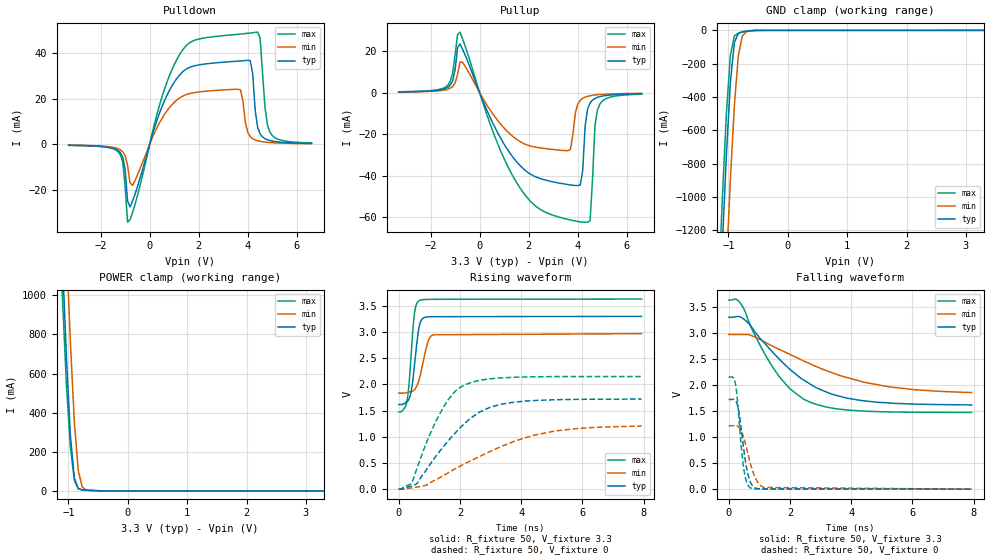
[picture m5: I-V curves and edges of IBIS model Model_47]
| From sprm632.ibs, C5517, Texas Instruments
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| Model based on original model for BC3350CTHYPU
|   Sub model PU_ON_COM_3P3
[model]   Model_47
|[Description]  [3.3V-I/O-PU-X, COM]
|   PU,COM,
|[Input Load]   PU
|[Output Drive]
|Voltage   3.3V
|Mode   I/O
Model_type   I/O
Polarity   Non-Inverting
Enable   Active-Low
Vinl =  0.8
Vinh =  2
Cref =  15.0000pF
Rref =  100.0000M
Vref =  0V
Vmeas =  1.65
C_comp   0.87673039p  0.86952386p   1.2993811p
[Model Spec]
Vinl   0.8   0.8   0.8
Vinh   2   2   2
[Temperature Range]   25   105   -10
[Voltage Range]   3.3   2.97   3.63
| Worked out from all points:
|   slope of the pulldown table from 0 to 0.495 V, typ, clamps not added: 30.2 ohm
|   slope of the pullup table from 0 to 0.495 V, typ, clamps not added: 36.2 ohm
|   GND clamp passes 1 mA (typ) near -0.58 V on its own axis
|   POWER clamp passes 1 mA (typ) near -0.52 V on its own axis
|   rising waveform, R_fixture 50, V_fixture 3.3: 20-80 % time 198ps typ, 268ps min, 165ps max; typ from 1.62 V to 3.3 V
|   rising waveform, R_fixture 50, V_fixture 0: 20-80 % time 1.53ns typ, 2.64ns min, 1.02ns max; typ from 0.002 V to 1.72 V
|   falling waveform, R_fixture 50, V_fixture 3.3: 20-80 % time 1.91ns typ, 2.84ns min, 1.38ns max; typ from 3.3 V to 1.62 V
|   falling waveform, R_fixture 50, V_fixture 0: 20-80 % time 244ps typ, 350ps min, 199ps max; typ from 1.72 V to 0.002 V
[POWER_clamp]
-3.3V     22.37A     22.96A     22.14A
-1.167V   1.737A     2.381A     1.512A
-1.1V     1.183A     1.806A     986.6mA
-1.033V   682.1mA    1.26A      542.1mA
-966.7mV  284.5mA    761.6mA    224.8mA
-900mV    65.81mA    352.3mA    53.51mA
-833.3mV  11.58mA    102.8mA    10.59mA
-766.7mV  4.716mA    20.06mA    5.567mA
-700mV    3.207mA    4.896mA    4.024mA
-633.3mV  2.25mA     2.24mA     2.841mA
3.3V      -103.5uA   -77.89uA   -144.3uA
[Pulldown]
-3.3V     -379.4uA   -332.5uA   -410.9uA
-1.2V     -3.537mA   -2.351mA   -4.45mA
-1V       -10.99mA   -4.979mA   -18.19mA
-900mV    -24.8mA    -9.223mA   -34.14mA
-700mV    -24.92mA   -18.03mA   -29.99mA
500mV     16.51mA    11.37mA    20.75mA
1.5V      33.12mA    21.9mA     43.48mA
3.7V      36.65mA    23.93mA    48.44mA
4.1V      36.79mA    3.426mA    48.89mA
4.4V      7.557mA    1.597mA    49.31mA
4.9V      1.707mA    822.5uA    5.402mA
6.6V      436uA      304.4uA    625.7uA
[Pullup]
-3.3V     352.6uA    285.2uA    404.5uA
-1.3V     2.559mA    1.632mA    3.524mA
-800mV    23.47mA    14.67mA    29.18mA
800mV     -20.79mA   -14.38mA   -26.49mA
2V        -38.75mA   -25.51mA   -51.47mA
3.7V      -44.51mA   -27.32mA   -61.38mA
4.2V      -37.5mA    -2.71mA    -62.46mA
4.3V      -15.99mA   -2.138mA   -62.46mA
4.5V      -4.997mA   -1.493mA   -61.74mA
4.7V      -2.803mA   -1.142mA   -15.75mA
4.9V      -1.928mA   -922.7uA   -5.515mA
6.6V      -515.4uA   -347uA     -755.5uA
[GND_clamp]
-3.3V     -22.52A    -23.16A    -22.27A
-1.167V   -1.839A    -2.548A    -1.554A
-1.1V     -1.269A    -1.966A    -993.7mA
-1.033V   -744.2mA   -1.409A    -496.6mA
-966.7mV  -312.7mA   -893.3mA   -149.2mA
-900mV    -73.61mA   -452.5mA   -34.27mA
-833.3mV  -18.5mA    -154mA     -16.8mA
-766.7mV  -8.937mA   -34.95mA   -10.26mA
-700mV    -4.785mA   -8.919mA   -5.557mA
-633.3mV  -2.174mA   -3.321mA   -2.412mA
3.3V      469pA      103.6uA    -29.49uA
[Ramp]
dV/dt_f  1.0208248/1.9222786n 0.68955168/2.9572302n  1.3051325/1.3845332n
dV/dt_r  1.0324428/1.5316798n 0.73040027/2.6850092n  1.2903206/1.0171168n
R_load = 50
[Rising Waveform]
R_fixture = 50
V_fixture = 3.3
V_fixture_min = 2.97
V_fixture_max = 3.63
0s        1.617V     1.835V     1.475V
258.2ps   1.665V     1.845V     1.646V
316.8ps   1.7V       1.852V     1.878V
381.2ps   1.797V     1.861V     2.348V
469.6ps   2.119V     1.879V     3.082V
523.7ps   2.41V      1.906V     3.389V
692.9ps   3.16V      2.15V      3.606V
955.9ps   3.29V      2.814V     3.624V
1.128ns   3.294V     2.948V     3.625V
7.933ns   3.3V       2.97V      3.63V
[Rising Waveform]
R_fixture = 50
V_fixture = 0
V_fixture_min = 0
V_fixture_max = 0
0s        2.331mV    2.258mV    2.773mV
416.9ps   60.92mV    27.58mV    119mV
604.9ps   116.9mV    43.18mV    412.1mV
1.347ns   731.5mV    223.8mV    1.445V
1.792ns   1.04V      373.7mV    1.838V
2.183ns   1.272V     493.9mV    1.998V
3.005ns   1.57V      726.5mV    2.109V
3.777ns   1.662V     915.7mV    2.138V
5.109ns   1.709V     1.112V     2.15V
7.933ns   1.721V     1.206V     2.152V
[Falling Waveform]
R_fixture = 50
V_fixture = 3.3
V_fixture_min = 2.97
V_fixture_max = 3.63
0s        3.3V       2.97V      3.63V
376.7ps   3.309V     2.97V      3.576V
903.3ps   2.983V     2.907V     2.9V
1.423ns   2.639V     2.747V     2.356V
1.986ns   2.306V     2.592V     1.934V
2.534ns   2.065V     2.439V     1.703V
3.338ns   1.83V      2.244V     1.561V
4.328ns   1.702V     2.069V     1.502V
6.052ns   1.634V     1.911V     1.477V
7.933ns   1.618V     1.857V     1.474V
[Falling Waveform]
R_fixture = 50
V_fixture = 0
V_fixture_min = 0
V_fixture_max = 0
0s        1.722V     1.218V     2.152V
188.3ps   1.719V     1.223V     2.097V
301.4ps   1.58V      1.206V     1.609V
413.9ps   1.144V     1.118V     798.3mV
504.2ps   713.5mV    967mV      349.3mV
623.6ps   300.3mV    689.7mV    85.27mV
737.1ps   105mV      432.7mV    19.52mV
928.5ps   13.85mV    152.6mV    6.355mV
1.136ns   5.824mV    33.89mV    5.172mV
7.933ns   1.739mV    1.445mV    2.093mV
